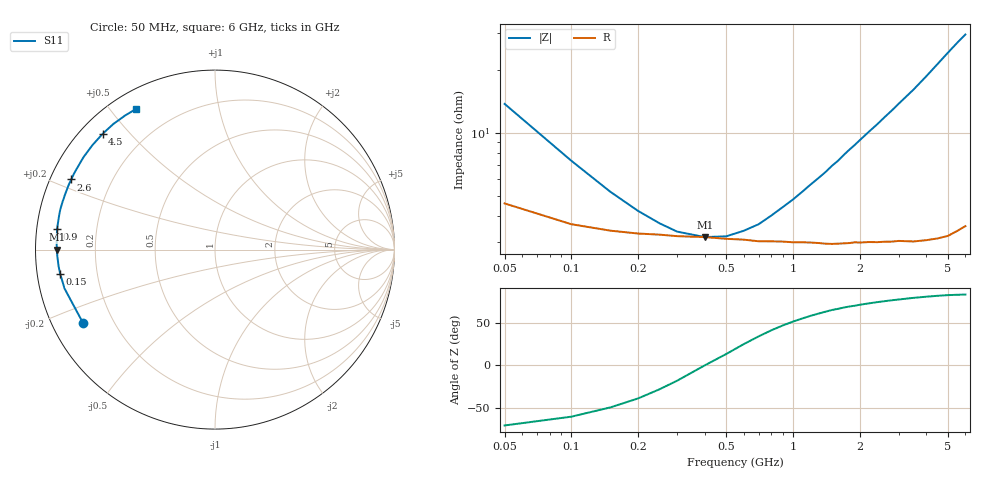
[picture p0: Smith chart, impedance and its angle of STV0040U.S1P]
! SIEMENS Discrete & RF Semiconductors
! BA892
! Si PIN Diode in SCD-80
! IF = 0.04 mA
! S-Parameters:  September  1997
# GHz  S  MA  R  50
!  f  S11
! GHz  MAG  ANG
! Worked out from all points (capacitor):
!   34 points, 50 MHz to 6 GHz, reference 50 ohm
!   read as one part to ground: C = 234 pF near 50 MHz
!   lowest |Z| = 3.18 ohm at 400 MHz (marker M1)
!   series resonance near 400 MHz, so ESL is about 680 pH
!   S11 on the Smith chart (normalised r, x): 50 MHz: 0.09, -0.26; 150 MHz: 0.07, -0.08; 900 MHz: 0.06, +0.06; 2.6 GHz: 0.06, +0.23; 4.5 GHz: 0.06, +0.42; 6 GHz: 0.07, +0.58
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0.05  0.8413 -150.8
0.1  0.8656 -165.4
0.15  0.873 -170.9
0.2  0.8763 -173.9
0.25  0.8775 -176.0
0.3  0.8793 -177.6
0.4  0.8804 -180.0
0.5  0.8826 178.3
0.6  0.8836 176.7
0.7  0.8857 175.3
0.8  0.8859 173.9
0.9  0.8863 172.6
1.2  0.888 169.0
1.4  0.8897 166.8
1.5  0.8902 165.6
1.6  0.8902 164.6
1.8  0.8901 162.3
2.2  0.8903 158.1
2.4  0.8911 156.1
2.6  0.8914 154.0
2.8  0.8922 152.0
3  0.8924 149.9
3.5  0.8955 144.9
4  0.8972 139.6
4.5  0.899 134.2
5  0.9003 128.9
5.5  0.8994 123.9
6  0.8985 119.3
